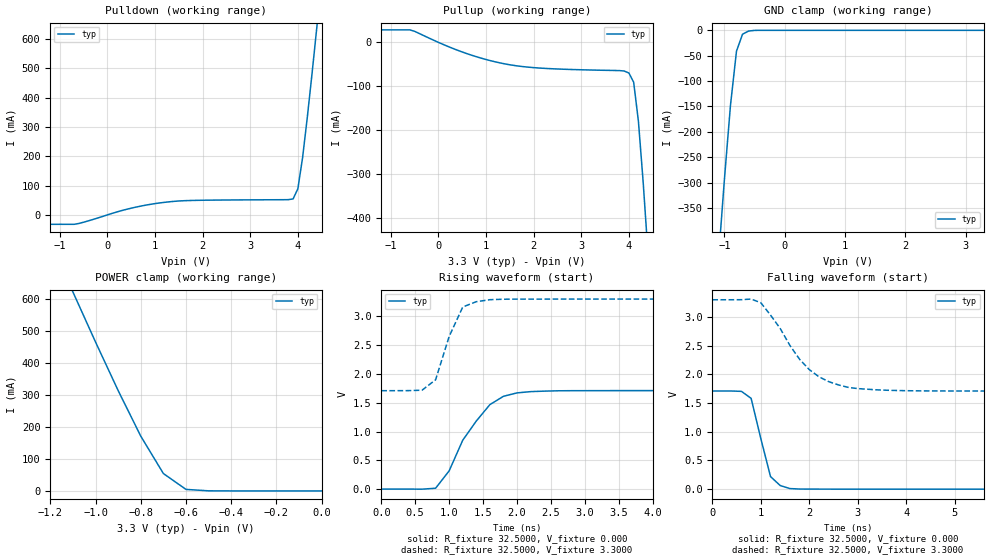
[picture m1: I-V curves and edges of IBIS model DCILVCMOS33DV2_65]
| / 7\'7
| \ \   Xilinx Inc.
| / /
| \_\/.\   IBIS Model for Virtex-II
[IBIS ver]   2.1
[File name]   dci3365d.ibs
[File Rev]   1.1
[Date]   Aug. 3, 2001
[Source]   Hspice simulations (08-03: TT, SS, FF)
[Notes]   Xilinx IBIS model for LVDCI 3.3V 32.5 ohms (65/2) driver
[Disclaimer] The data in this model is derived from SPICE simulations using
   modeling information extracted from the target process. While
   a great deal of care has been taken to provide information
   that is accurate, this model is considered preliminary as it
   has not been verified by actual silicon measurement. Treat the
   data in this model as preliminary until actual silicon
   verification is performed.
[Copyright]   Copyright 2001, Xilinx Inc., All rights reserved
|   Component Virtex_II
[Component]   Virtex_II
[Manufacturer]   Xilinx Inc.
[Package]
| variable   typ   min   max
R_pkg   0.1000   NA   NA
L_pkg   0.8000nH   NA   NA
C_pkg   0.5000pF   NA   NA
[Pin]  signal_name   model_name   R_pin   L_pin   C_pin
io   DCILVCMOS33DV2_65   DCILVCMOS33DV2_65
| ins  insig   inp
| ens  ensig   inp
PGND   GND   GND
VCCO   VCCO   POWER
| Models and submodels in the file (1): DCILVCMOS33DV2_65 (I/O)
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|   Model DCILVCMOS33DV2_65
[Model]   DCILVCMOS33DV2_65
Model_type   I/O
Polarity   Non-Inverting
Enable   Active-Low
Vinh = 2.0V
Vinl = 0.8V
Vmeas =   1.4000V
Cref =  35.0000pF
Rref =   1.0000M
Vref =  0.000V
C_comp   7.0000pF   NA   NA
[Temperature Range]   25.0000   NA   NA
[Voltage Range]   3.3000V   NA   NA
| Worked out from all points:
|   slope of the pulldown table from 0 to 0.495 V, typ, clamps not added: 21.8 ohm
|   slope of the pullup table from 0 to 0.495 V, typ, clamps not added: 22.8 ohm
|   GND clamp passes 1 mA (typ) near -0.57 V on its own axis
|   POWER clamp passes 1 mA (typ) near -0.52 V on its own axis
|   rising waveform, R_fixture 32.5000, V_fixture 0.000: 20-80 % time 521ps typ, NA min, NA max; typ from 0 V to 1.71 V
|   rising waveform, R_fixture 32.5000, V_fixture 3.3000: 20-80 % time 295ps typ, NA min, NA max; typ from 1.71 V to 3.3 V
|   falling waveform, R_fixture 32.5000, V_fixture 0.000: 20-80 % time 302ps typ, NA min, NA max; typ from 1.71 V to 0 V
|   falling waveform, R_fixture 32.5000, V_fixture 3.3000: 20-80 % time 845ps typ, NA min, NA max; typ from 3.3 V to 1.71 V
[Pulldown]
| voltage   I(typ)   I(min)   I(max)
-3.3V     -32.11mA   NA         NA
-700mV    -32.11mA   NA         NA
500mV     22.88mA    NA         NA
1.2V      42.83mA    NA         NA
1.8V      49.32mA    NA         NA
3.9V      54.53mA    NA         NA
4V        89.07mA    NA         NA
4.1V      196.2mA    NA         NA
4.2V      335.2mA    NA         NA
4.3V      485.2mA    NA         NA
4.5V      799.3mA    NA         NA
6.6V      4.271A     NA         NA
[Pullup]
| voltage   I(typ)   I(min)   I(max)
-3.3V     28.49mA    NA         NA
-600mV    28.49mA    NA         NA
500mV     -21.9mA    NA         NA
1.4V      -49.12mA   NA         NA
2.2V      -59.01mA   NA         NA
3.9V      -65.23mA   NA         NA
4V        -69.8mA    NA         NA
4.1V      -90.79mA   NA         NA
4.2V      -179.8mA   NA         NA
4.3V      -319mA     NA         NA
4.5V      -638.9mA   NA         NA
6.6V      -4.321A    NA         NA
[GND_clamp]
| voltage   I(typ)   I(min)   I(max)
-3.3V     -4.301A    NA         NA
-1.1V     -452.1mA   NA         NA
-1V       -293.4mA   NA         NA
-900mV    -148.1mA   NA         NA
-800mV    -41.07mA   NA         NA
-700mV    -7.668mA   NA         NA
-600mV    -1.449mA   NA         NA
-400mV    -8.141uA   NA         NA
3.3V      540.8nA    NA         NA
[POWER_clamp]
| voltage   I(typ)   I(min)   I(max)
-3.3V     4.254A     NA         NA
-1.1V     621.4mA    NA         NA
-1V       465.1mA    NA         NA
-900mV    313.6mA    NA         NA
-800mV    171.2mA    NA         NA
-700mV    54.37mA    NA         NA
-600mV    4.797mA    NA         NA
-500mV    289.2uA    NA         NA
0V        540.8nA    NA         NA
[Ramp]
| variable   typ   min   max
dV/dt_r   1.0260/0.4491n   NA   NA
dV/dt_f   0.9546/0.7976n   NA   NA
R_load = 32.5000
[Rising Waveform]
R_fixture = 32.5000
V_fixture = 0.000
| time   V(typ)   V(min)   V(max)
0s        8.575uV    NA         NA
800ps     14.81mV    NA         NA
1ns       317.1mV    NA         NA
1.2ns     848.6mV    NA         NA
1.4ns     1.182V     NA         NA
1.6ns     1.466V     NA         NA
1.8ns     1.611V     NA         NA
2ns       1.671V     NA         NA
2.8ns     1.709V     NA         NA
10ns      1.71V      NA         NA
[Rising Waveform]
R_fixture = 32.5000
V_fixture = 3.3000
V_fixture_min = 3.0000
V_fixture_max = 3.6000
| time   V(typ)   V(min)   V(max)
0s        1.709V     NA         NA
600ps     1.717V     NA         NA
800ps     1.898V     NA         NA
1ns       2.651V     NA         NA
1.2ns     3.162V     NA         NA
1.4ns     3.255V     NA         NA
1.6ns     3.289V     NA         NA
1.8ns     3.297V     NA         NA
2.6ns     3.3V       NA         NA
10ns      3.3V       NA         NA
[Falling Waveform]
R_fixture = 32.5000
V_fixture = 0.000
| time   V(typ)   V(min)   V(max)
0s        1.71V      NA         NA
600ps     1.704V     NA         NA
800ps     1.582V     NA         NA
1ns       881.1mV    NA         NA
1.2ns     219.4mV    NA         NA
1.4ns     63.12mV    NA         NA
1.6ns     10.7mV     NA         NA
1.8ns     2.152mV    NA         NA
2.4ns     564.4uV    NA         NA
10ns      1.487uV    NA         NA
[Falling Waveform]
R_fixture = 32.5000
V_fixture = 3.3000
V_fixture_min = 3.0000
V_fixture_max = 3.6000
| time   V(typ)   V(min)   V(max)
0s        3.3V       NA         NA
800ps     3.312V     NA         NA
1ns       3.248V     NA         NA
1.4ns     2.799V     NA         NA
1.8ns     2.263V     NA         NA
2ns       2.083V     NA         NA
2.4ns     1.873V     NA         NA
2.8ns     1.774V     NA         NA
4.2ns     1.713V     NA         NA
10ns      1.709V     NA         NA
